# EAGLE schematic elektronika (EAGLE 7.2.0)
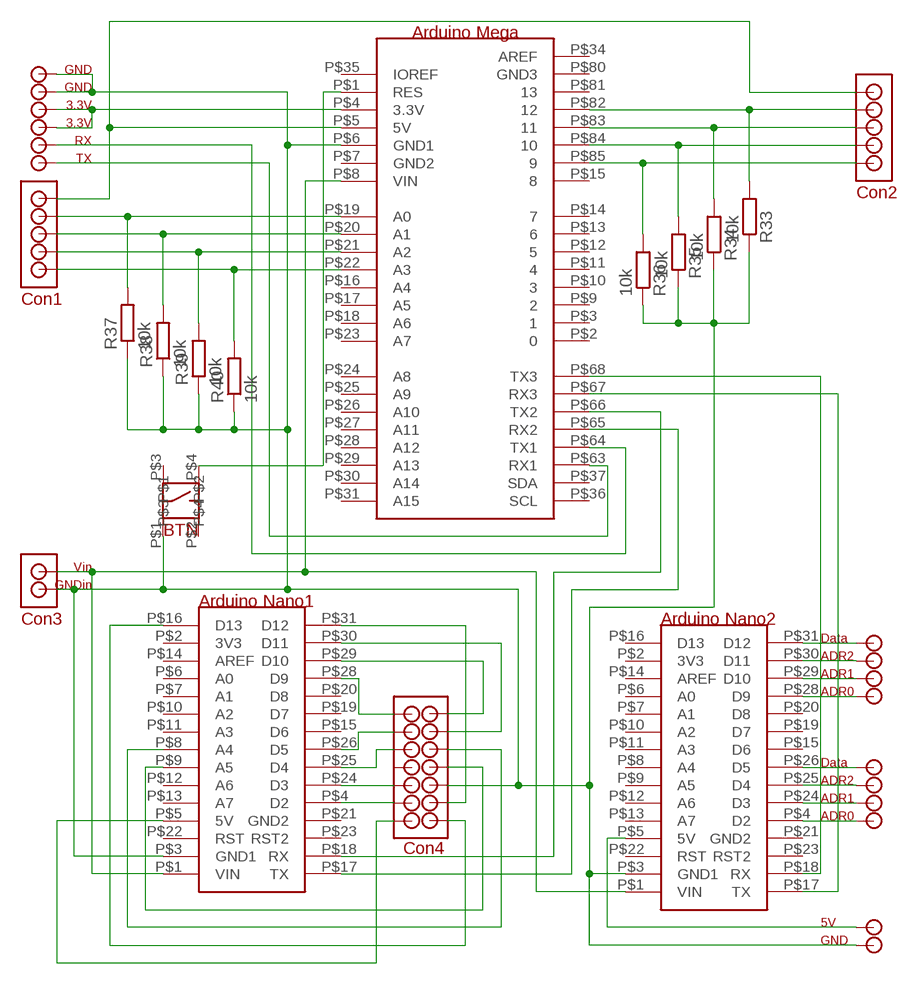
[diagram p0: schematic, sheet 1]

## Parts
R33  10k  R-EU_R1206  [R1206]
R34  10k  R-EU_R1206  [R1206]
R35  10k  R-EU_R1206  [R1206]
R36  10k  R-EU_R1206  [R1206]
R37  10k  R-EU_R1206  [R1206]
R38  10k  R-EU_R1206  [R1206]
R39  10k  R-EU_R1206  [R1206]
R40  10k  R-EU_R1206  [R1206]
U$4  NANO  [NANO]
U$5  NANO  [NANO]
U$14  MEGA  [MEGA]
U$15  CON_1  [CON_1]
U$16  Data  CON_1  [CON_1]
U$18  ADR0  CON_1  [CON_1]
U$21  ADR1  CON_1  [CON_1]
U$22  ADR2  CON_1  [CON_1]
U$23  Data  CON_1  [CON_1]
U$32  ADR0  CON_1  [CON_1]
U$33  ADR1  CON_1  [CON_1]
U$34  ADR2  CON_1  [CON_1]
U$35  5V  CON_1  [CON_1]
U$36  GND  CON_1  [CON_1]
U$38  CON_1  [CON_1]
U$39  CON_1  [CON_1]
U$42  CON_1  [CON_1]
U$43  CON_1  [CON_1]
U$46  CON_1  [CON_1]
U$47  CON_1  [CON_1]
U$50  CON_1  [CON_1]
U$51  CON_1  [CON_1]
U$52  CON_1  [CON_1]
U$53  CON_1  [CON_1]
U$54  CON_1  [CON_1]
U$55  CON_1  [CON_1]
U$56  CON_1  [CON_1]
U$57  3.3V  CON_1  [CON_1]
U$58  3.3V  CON_1  [CON_1]
U$59  GND  CON_1  [CON_1]
U$60  GND  CON_1  [CON_1]
U$61  RX  CON_1  [CON_1]
U$62  TX  CON_1  [CON_1]
U$63  GNDin  CON_1  [CON_1]
U$65  BUTTON  [BUT]
U$66  Vin  CON_1  [CON_1]
U$68  CON_1  [CON_1]
U$69  CON_1  [CON_1]
U$70  CON_1  [CON_1]
U$71  CON_1  [CON_1]
U$72  CON_1  [CON_1]
U$73  CON_1  [CON_1]
U$74  CON_1  [CON_1]
U$75  CON_1  [CON_1]
U$76  CON_1  [CON_1]
U$77  CON_1  [CON_1]

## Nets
N$1: R37.2 U$14.P$19(A0) U$73.P$1
N$2: R38.2 U$14.P$20(A1) U$75.P$1
N$3: R39.2 U$14.P$21(A2) U$76.P$1
N$5: R33.1 R34.1 R35.1 R36.1 R37.1 R38.1 R39.1 R40.1 U$4.P$3(GND1) U$5.P$3(GND1) U$14.P$6(GND1) U$36.P$1 U$53.P$1 U$59.P$1 U$60.P$1 U$63.P$1 U$65.P$1
N$6: R33.2 U$14.P$82 U$68.P$1
N$7: U$5.P$18(RX) U$14.P$66(TX2)
N$8: U$4.P$1(VIN) U$5.P$1(VIN) U$14.P$8(VIN) U$66.P$1
N$9: R35.2 U$14.P$84 U$71.P$1
N$10: U$5.P$31(D12) U$46.P$1
N$11: U$5.P$30(D11) U$47.P$1
N$20: R40.2 U$14.P$22(A3) U$77.P$1
N$21: U$5.P$29(D10) U$50.P$1
N$32: U$4.P$30(D11) U$34.P$1
N$42: U$5.P$28(D9) U$51.P$1
N$52: U$5.P$16(D13) U$43.P$1
N$58: U$14.P$1(RES) U$65.P$4
N$61: U$4.P$31(D12) U$23.P$1
N$62: U$4.P$25(D4) U$22.P$1
N$63: U$4.P$28(D9) U$32.P$1
N$64: U$4.P$29(D10) U$33.P$1
N$66: U$5.P$25(D4) U$42.P$1
N$67: U$5.P$26(D5) U$39.P$1
N$68: U$5.P$24(D3) U$38.P$1
N$69: U$5.P$8(A4) U$54.P$1
N$70: U$5.P$9(A5) U$55.P$1
N$71: U$5.P$4(D2) U$56.P$1
N$72: U$5.P$5(5V) U$52.P$1
N$73: U$4.P$26(D5) U$16.P$1
N$78: U$5.P$17(TX) U$14.P$65(RX2)
N$80: U$4.P$18(RX) U$14.P$68(TX3)
N$81: U$4.P$17(TX) U$14.P$67(RX3)
N$83: U$4.P$24(D3) U$21.P$1
N$84: U$4.P$4(D2) U$18.P$1
N$86: R34.2 U$14.P$83 U$70.P$1
N$88: R36.2 U$14.P$85 U$72.P$1
N$90: U$14.P$4(3.3V) U$57.P$1 U$58.P$1
N$91: U$14.P$5(5V) U$69.P$1 U$74.P$1
N$92: U$14.P$63(RX1) U$62.P$1
N$93: U$14.P$64(TX1) U$61.P$1
N$95: U$4.P$5(5V) U$35.P$1
Unconnected: U$4.P$2(3V3) U$4.P$6(A0) U$4.P$7(A1) U$4.P$8(A4) U$4.P$9(A5) U$4.P$10(A2) U$4.P$11(A3) U$4.P$12(A6) U$4.P$13(A7) U$4.P$14(AREF) U$4.P$15(D6) U$4.P$16(D13) U$4.P$19(D7) U$4.P$20(D8) U$4.P$21(GND2) U$4.P$22(RST) U$4.P$23(RST2) U$5.P$2(3V3) U$5.P$6(A0) U$5.P$7(A1) U$5.P$10(A2) U$5.P$11(A3) U$5.P$12(A6) U$5.P$13(A7) U$5.P$14(AREF) U$5.P$15(D6) U$5.P$19(D7) U$5.P$20(D8) U$5.P$21(GND2) U$5.P$22(RST) U$5.P$23(RST2) U$14.P$2 U$14.P$3 U$14.P$7(GND2) U$14.P$9 U$14.P$10 U$14.P$11 U$14.P$12 U$14.P$13 U$14.P$14 U$14.P$15 U$14.P$16(A4) U$14.P$17(A5) U$14.P$18(A6) U$14.P$23(A7) U$14.P$24(A8) U$14.P$25(A9) U$14.P$26(A10) U$14.P$27(A11) U$14.P$28(A12) U$14.P$29(A13) U$14.P$30(A14) U$14.P$31(A15) U$14.P$34(AREF) U$14.P$35(IOREF) U$14.P$36(SCL) U$14.P$37(SDA) U$14.P$80(GND3) U$14.P$81 U$15.P$1 U$65.P$2 U$65.P$3

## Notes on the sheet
- Arduino Mega
- Con2
- Con1
- BTN
- Arduino Nano1
- Con3 | Arduino Nano2
- Con4

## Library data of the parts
R33-R40 = rcl:R-EU_: RESISTOR, European symbol
U$4 U$5 = arduino:NANO
U$14 = arduino:MEGA
U$15 U$16 U$18 U$21-U$23 U$32-U$36 U$38 U$39 U$42 U$43 U$46 U$47 U$50-U$63 U$66 U$68-U$77 = arduino:CON_1
U$65 = arduino:BUTTON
